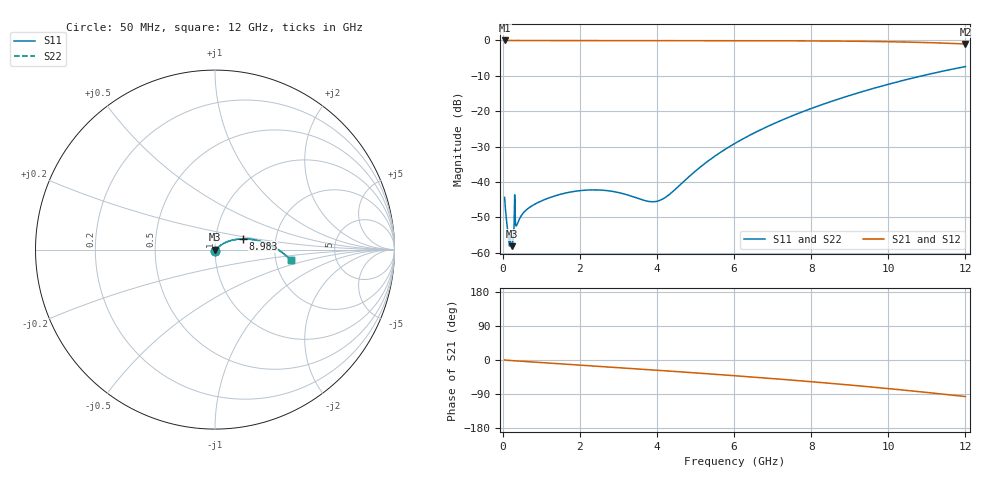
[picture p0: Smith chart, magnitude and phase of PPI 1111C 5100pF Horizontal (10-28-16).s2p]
# MHz S MA R 50
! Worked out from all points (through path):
!   1601 points, 50 MHz to 12 GHz, reference 50 ohm
!   highest |S21| = 0.00 dB at 50 MHz (marker M1); lowest = -1.0 dB at 12 GHz (marker M2)
!   group delay of S21, straight-line fit = 21.8 ps
!   lowest |S11| = -58.1 dB at 229.2 MHz (marker M3), VSWR 1.00, Z = 50.1 - j0.059 ohm
!   |S11| at or under -10 dB: start of sweep to 10.87 GHz
!   |S22| runs from -58.1 to -7.4 dB; largest |S21 - S12| = 0
!   S11 on the Smith chart (normalised r, x): 50 MHz: 1.00, -0.01; 8.983 GHz: 1.35, +0.17; 12 GHz: 2.43, -0.36
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50  0.006096 -86.6  0.9996 0.0  0.9996 0.0  0.006096 -86.6
124.6875  0.002154 -75.9  0.9994 -0.7  0.9994 -0.7  0.002154 -75.9
162.0312  0.001434 -61.3  0.9993 -1.0  0.9993 -1.0  0.001434 -61.3
199.375  0.001683 -46.3  0.9988 -1.3  0.9988 -1.3  0.001683 -46.3
229.25  0.001245 -28.2  0.9989 -1.5  0.9989 -1.5  0.001245 -28.2
259.125  0.001405 -5.6  0.9986 -1.8  0.9986 -1.8  0.001405 -5.6
356.2188  0.002411 -23.5  0.9977 -2.4  0.9977 -2.4  0.002411 -23.5
393.5625  0.002682 -18.1  0.9974 -2.7  0.9974 -2.7  0.002682 -18.1
520.5312  0.003588 -23.8  0.9966 -3.5  0.9966 -3.5  0.003588 -23.8
677.375  0.004316 -34.0  0.9962 -4.5  0.9962 -4.5  0.004316 -34.0
1297.281  0.006239 -56.6  0.9957 -8.6  0.9957 -8.6  0.006239 -56.6
2044.156  0.007608 -67.5  0.9954 -13.6  0.9954 -13.6  0.007608 -67.5
2761.156  0.00751 -68.9  0.995 -18.4  0.995 -18.4  0.00751 -68.9
3754.5  0.005374 -39.7  0.9946 -25.2  0.9946 -25.2  0.005374 -39.7
4038.312  0.005425 -16.8  0.9944 -27.2  0.9944 -27.2  0.005425 -16.8
4322.125  0.006684 5.8  0.9943 -29.2  0.9943 -29.2  0.006684 5.8
5308  0.01948 35.8  0.9935 -36.2  0.9935 -36.2  0.01948 35.8
6025  0.03523 37.9  0.9926 -41.5  0.9926 -41.5  0.03523 37.9
8019.156  0.1103 28.5  0.9856 -57.4  0.9856 -57.4  0.1103 28.5
8982.625  0.166 21.1  0.9769 -65.9  0.9769 -65.9  0.166 21.1
10013.31  0.2414 12.1  0.9601 -75.6  0.9601 -75.6  0.2414 12.1
12000  0.428 -8.0  0.8912 -96.4  0.8912 -96.4  0.428 -8.0
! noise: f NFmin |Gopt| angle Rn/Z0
50  0.0004124  0.8783  0.3465  0.0007331
1372  0.007352  0.8197  9.404  0.008486
2701  0.0109  0.771  18.38  0.009468
4031  0.01396  0.7443  27.1  0.01037
5360  0.01683  0.7304  35.45  0.01131
6682  0.01965  0.7256  43.31  0.01234
8012  0.02257  0.7276  50.73  0.01353
9341  0.02566  0.7349  57.66  0.01494
1.067e+04  0.029  0.7464  64.09  0.01666
1.2e+04  0.03271  0.761  70.05  0.01878
